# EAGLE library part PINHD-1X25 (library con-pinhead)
PIN HEADER
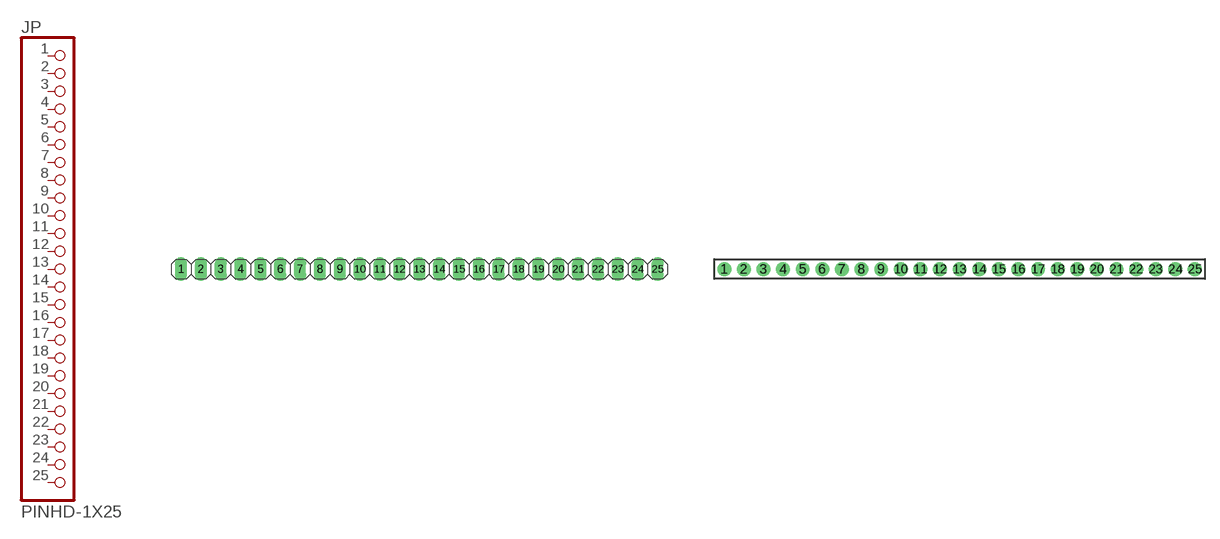
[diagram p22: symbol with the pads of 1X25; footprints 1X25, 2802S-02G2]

Designator prefix JP

## PINHD-1X25_2.54  [1X25]
1  1  pas
2  2  pas
3  3  pas
4  4  pas
5  5  pas
6  6  pas
7  7  pas
8  8  pas
9  9  pas
10  10  pas
11  11  pas
12  12  pas
13  13  pas
14  14  pas
15  15  pas
16  16  pas
17  17  pas
18  18  pas
19  19  pas
20  20  pas
21  21  pas
22  22  pas
23  23  pas
24  24  pas
25  25  pas

## PINHD-1X25_2802S-02G2  [2802S-02G2]
Pads as for 1X25

## PINHD-1X25_2.00  [1X25M]
Pads as for 1X25

## PINHD-1X25_2.54-90°  [1X25/90]
Pads as for 1X25

## PINHD-1X25_2.54-SMD  [1X25SMD]
Pads as for 1X25

## PINHD-1X25_2.54-SMD-90°  [1X25SMD/90]
Pads as for 1X25

## Footprint 1X25 (pad centres in mm)
PIN HEADER - 2.54
drill 1.016 long: 1 -29.21,0; 2 -26.67,0; 3 -24.13,0; 4 -21.59,0; 5 -19.05,0; 6 -16.51,0; 7 -13.97,0; 8 -11.43,0; 9 -8.89,0; 10 -6.35,0; 11 -3.81,0; 12 -1.27,0; 13 1.27,0; 14 3.81,0; 15 6.35,0; 16 8.89,0; 17 11.43,0; 18 13.97,0; 19 16.51,0; 20 19.05,0; 21 21.59,0; 22 24.13,0; 23 26.67,0; 24 29.21,0; 25 31.75,0

## Footprint 2802S-02G2 (pad centres in mm)
2mm Center - .020 inch Square Pin - Single Row Straight Header Source: http://www.commcon.com/main
drill 0.8 pad 1.422: 1 -24,0; 2 -22,0; 3 -20,0; 4 -18,0; 5 -16,0; 6 -14,0; 7 -12,0; 8 -10,0; 9 -8,0; 10 -6,0; 11 -4,0; 12 -2,0; 13 0,0; 14 2,0; 15 4,0; 16 6,0; 17 8,0; 18 10,0; 19 12,0; 20 14,0; 21 16,0; 22 18,0; 23 20,0; 24 22,0; 25 24,0

## Footprint 1X25M (pad centres in mm)
PIN HEADER - 2
drill 0.914 square: 1 -24,0
drill 0.914: 2 -22,0; 3 -20,0; 4 -18,0; 5 -16,0; 6 -14,0; 7 -12,0; 8 -10,0; 9 -8,0; 10 -6,0; 11 -4,0; 12 -2,0; 13 0,0; 14 2,0; 15 4,0; 16 6,0; 17 8,0; 18 10,0; 19 12,0; 20 14,0; 21 16,0; 22 18,0; 23 20,0; 24 22,0; 25 24,0

## Footprint 1X25/90 (pad centres in mm)
PIN HEADER - 2.54 90°
drill 1.016 long: 1 -24.13,-3.81; 2 -21.59,-3.81; 3 -19.05,-3.81; 4 -16.51,-3.81; 5 -13.97,-3.81; 6 -11.43,-3.81; 7 -8.89,-3.81; 8 -6.35,-3.81; 9 -3.81,-3.81; 10 -1.27,-3.81; 11 1.27,-3.81; 12 3.81,-3.81; 13 6.35,-3.81; 14 8.89,-3.81; 15 11.43,-3.81; 16 13.97,-3.81; 17 16.51,-3.81; 18 19.05,-3.81; 19 21.59,-3.81; 20 24.13,-3.81; 21 26.67,-3.81; 22 29.21,-3.81; 23 31.75,-3.81; 24 34.29,-3.81; 25 36.83,-3.81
